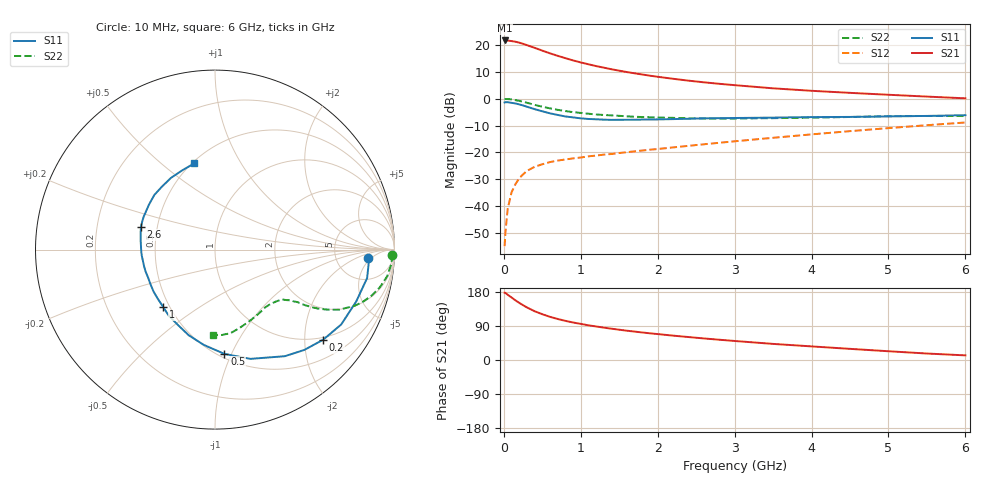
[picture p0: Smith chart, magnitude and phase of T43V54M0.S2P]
! Infineon Technologies  Discrete & RF Semiconductors
! BFR182T
! Si NPN RF Bipolar Junction Transistor in SC75
! VCE = 3.5 V  IC = 4 mA
! Common Emitter S-Parameters:  October  1999
# GHz  S  MA  R  50
!  f  S11  S21  S12  S22
! GHz  MAG  ANG  MAG  ANG  MAG  ANG  MAG  ANG
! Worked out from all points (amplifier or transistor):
!   36 points, 10 MHz to 6 GHz, reference 50 ohm
!   highest |S21| = 21.7 dB at 10 MHz (marker M1)
!   |S21| within 3 dB of that: start of sweep to 424.8 MHz
!   unconditionally stable (mu >= 1): 1.558 GHz to 4.101 GHz
!   at 250 MHz: K = 0.23, MSG = 24.3 dB, |S12| = -28.2 dB
!   at 1.4 GHz: K = 0.96, MSG = 15.8 dB, |S12| = -20.6 dB
!   at 6 GHz: K = 0.83, MSG = 4.5 dB, |S12| = -8.8 dB
!   S11 on the Smith chart (normalised r, x): 10 MHz: 11, -4; 200 MHz: 0.94, -2.45; 500 MHz: 0.53, -0.94; 1 GHz: 0.46, -0.36; 2.6 GHz: 0.40, +0.13; 6 GHz: 0.51, +0.65
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0.01  0.8538 -3.2  12.15 177.7  0.0018 83.8  0.9854 -1.7
0.02  0.8609 -2.9  12.08 177.1  0.0032 102.7  0.9877 -1.8
0.05  0.8622 -10.6  12.13 172.2  0.0089 87.5  0.9863 -4.5
0.1  0.8382 -20.2  11.83 165.0  0.0181 80.9  0.9708 -8.8
0.15  0.8176 -30.7  11.52 157.5  0.0255 74.3  0.9428 -12.8
0.2  0.7844 -39.8  11.07 150.8  0.0332 71.2  0.9113 -16.2
0.25  0.7485 -48.3  10.52 144.6  0.0391 66.3  0.8754 -19.3
0.3  0.7099 -56.8  9.943 138.8  0.0453 63.4  0.8404 -21.8
0.4  0.6401 -72.0  8.866 128.7  0.054 57.6  0.7693 -25.8
0.5  0.5836 -84.8  7.859 120.8  0.0603 54.4  0.7109 -28.1
0.6  0.5346 -96.7  6.999 113.9  0.0662 52.2  0.6618 -29.8
0.7  0.4993 -107.0  6.289 108.3  0.0705 50.9  0.6212 -30.9
0.8  0.4678 -116.3  5.691 103.3  0.0741 49.8  0.5892 -31.7
1  0.431 -132.0  4.733 95.3  0.0804 49.9  0.5444 -32.5
1.1  0.4199 -139.7  4.373 91.5  0.0846 50.3  0.5258 -33.3
1.6  0.406 -167.1  3.134 77.3  0.1012 53.0  0.4703 -36.3
2.2  0.4174 172.9  2.351 64.3  0.124 56.7  0.4405 -42.0
2.6  0.4316 163.0  2.021 56.9  0.1419 58.6  0.4294 -46.6
3.5  0.4451 145.8  1.562 42.5  0.1874 60.2  0.4348 -58.2
4.5  0.4585 130.3  1.286 29.4  0.2492 58.9  0.4571 -72.3
5.5  0.4784 112.2  1.096 17.1  0.3216 54.9  0.4775 -85.4
6  0.4935 103.5  1.017 12.2  0.3611 51.7  0.4759 -91.1
